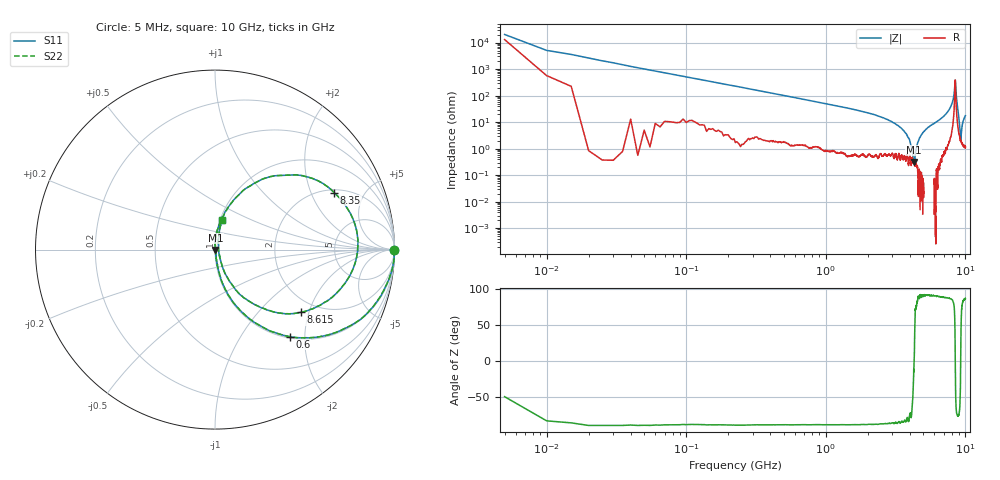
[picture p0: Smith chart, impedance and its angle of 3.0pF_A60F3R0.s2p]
! Amotech Co.,Ltd.
! http://www.amotech.co.kr/
! Part Number: A60F3R0
! These Parameters are Measured in Series Mode Connection
! Operation Temp=25[degC], DC Bias Voltage=0[V]
! Freq. Start=5[MHz] Stop=10[GHz], 2000[Steps]
! Date: Monday, July 20, 2020, 03:55:24
# GHZ S RI R 50.000000
!Freq.(Hz) S11(Real) S11(Imag) S21(Real) S21(Imag) S12(Real) S12(Imag) S22(Real) S22(Imag)
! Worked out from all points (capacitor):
!   2000 points, 5 MHz to 10 GHz, reference 50 ohm
!   read as one part in series: C = 3.16 pF near 55 MHz
!   lowest |Z| = 316 mohm at 4.25 GHz (marker M1)
!   series resonance near 4.296 GHz, so ESL is about 430 pH
!   S11 on the Smith chart (normalised r, x): 5 MHz: open; 600 MHz: 1.03, -1.69; 8.35 GHz: 2.14, +2.97; 8.615 GHz: 1.64, -1.77; 10 GHz: 1.02, +0.35
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0.005  0.9968 -0.00377  0.00319 0.00377  0.00319 0.00377  0.9968 -0.00377
0.065  0.9826 -0.1266  0.0174 0.1266  0.0174 0.1266  0.9826 -0.1266
0.145  0.9216 -0.2608  0.0784 0.2608  0.0784 0.2608  0.9216 -0.2608
0.32  0.7129 -0.4438  0.2871 0.4438  0.2871 0.4438  0.7129 -0.4438
0.6  0.4165 -0.4853  0.5835 0.4853  0.5835 0.4853  0.4165 -0.4853
1.675  0.0779 -0.2586  0.9221 0.2586  0.9221 0.2586  0.0779 -0.2586
3.34  0.0113 -0.0678  0.9887 0.0678  0.9887 0.0678  0.0113 -0.0678
3.96  0.00499 -0.0226  0.995 0.0226  0.995 0.0226  0.00499 -0.0226
4.14  0.00399 -0.0104  0.996 0.0104  0.996 0.0104  0.00399 -0.0104
4.25  0.00276 -0.00153  0.9972 0.00153  0.9972 0.00153  0.00276 -0.00153
4.56  0.00157 0.0173  0.9984 -0.0173  0.9984 -0.0173  0.00157 0.0173
5.005  0.00234 0.0425  0.9977 -0.0425  0.9977 -0.0425  0.00234 0.0425
6.67  0.0215 0.1317  0.9785 -0.1317  0.9785 -0.1317  0.0215 0.1317
7.88  0.155 0.3281  0.845 -0.3281  0.845 -0.3281  0.155 0.3281
8.335  0.6355 0.3441  0.3645 -0.3441  0.3645 -0.3441  0.6355 0.3441
8.35  0.6641 0.3179  0.3359 -0.3179  0.3359 -0.3179  0.6641 0.3179
8.465  0.7944 -0.00881  0.2056 0.00881  0.2056 0.00881  0.7944 -0.00881
8.615  0.4769 -0.3495  0.5231 0.3495  0.5231 0.3495  0.4769 -0.3495
8.84  0.1197 -0.2284  0.8803 0.2284  0.8803 0.2284  0.1197 -0.2284
9.25  0.0197 -0.00205  0.9803 0.00205  0.9803 0.00205  0.0197 -0.00205
9.53  0.0213 0.0816  0.9787 -0.0816  0.9787 -0.0816  0.0213 0.0816
10  0.0404 0.1661  0.9596 -0.1661  0.9596 -0.1661  0.0404 0.1661
